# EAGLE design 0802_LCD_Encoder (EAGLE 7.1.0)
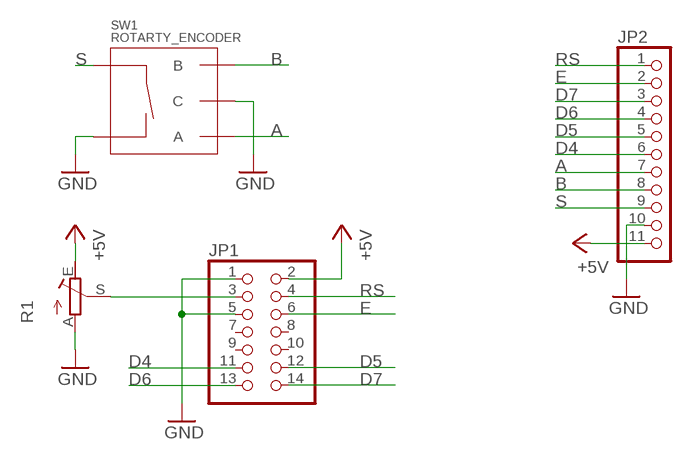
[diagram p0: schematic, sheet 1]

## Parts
JP1  PINHD-2X7  [2X07]
JP2  PINHD-1X11/90  [1X11/90]
R1  3302-TRIMMER  [3302-TRIMMER]
SW1  ROTARTY_ENCODER  [ROTARY_ENC_PLAIN]

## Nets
+5V: JP1.2 JP2.11 R1.E
A: JP2.7 SW1.A
B: JP2.8 SW1.B
D4: JP1.11 JP2.6
D5: JP1.12 JP2.5
D6: JP1.13 JP2.4
D7: JP1.14 JP2.3
E: JP1.6 JP2.2
GND: JP1.1 JP1.5 JP2.10 R1.A SW1.C SW1.SW-
RS: JP1.4 JP2.1
S: JP2.9 SW1.SW+
V0: JP1.3 R1.S
Unconnected: JP1.7 JP1.8 JP1.9 JP1.10

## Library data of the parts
JP1 = pinhead:PINHD-2X7: PIN HEADER
JP2 = pinhead:PINHD-1X11: PIN HEADER
R1 = 1Axel:3302-TRIMMER
SW1 = SparkFun-Electromechanical:ROTARTY_ENCODER: Simple no LED rotary encoder Example: COM-09117

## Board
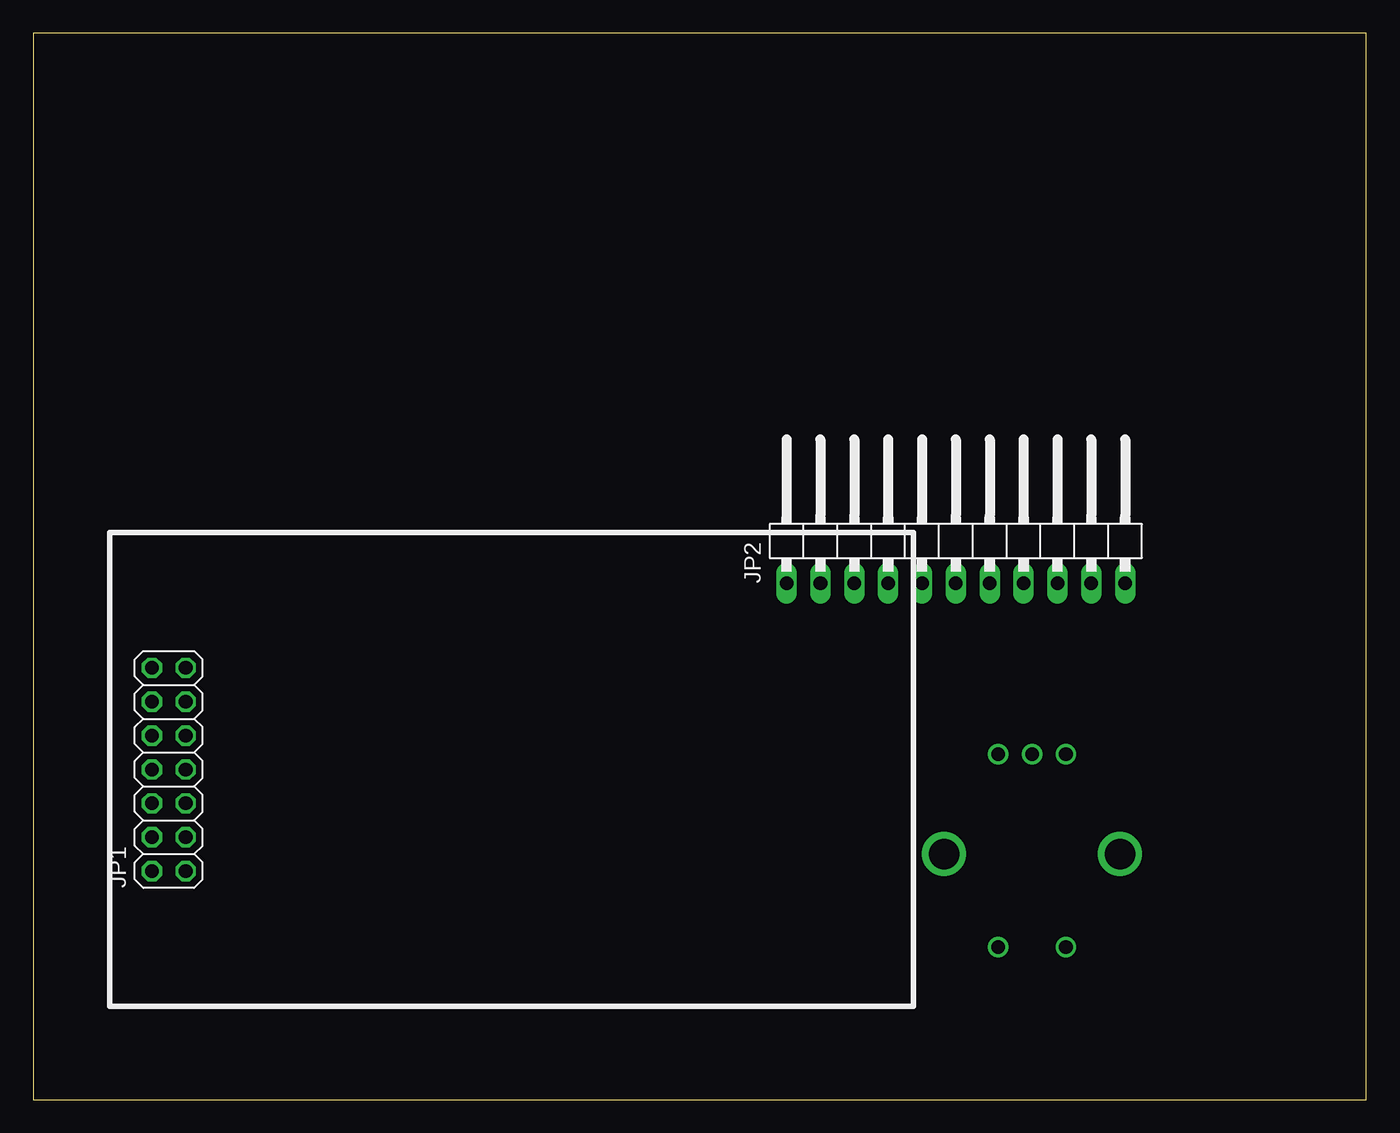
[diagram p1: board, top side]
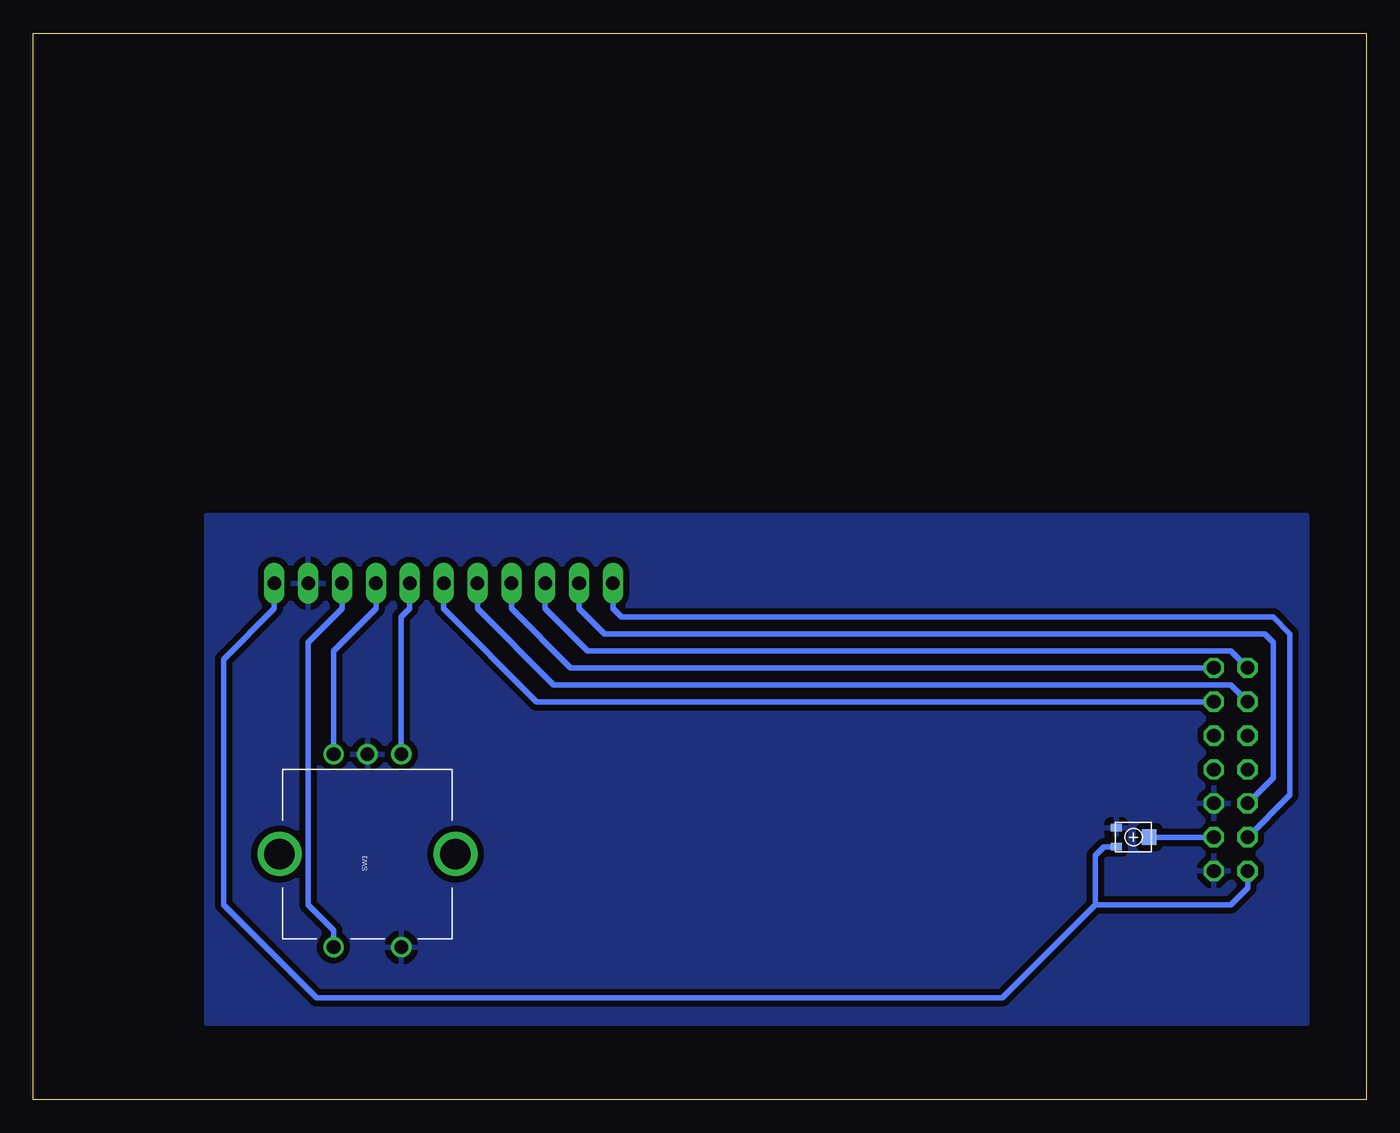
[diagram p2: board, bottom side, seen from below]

Size 100 x 80 mm. Coordinates in mm from the lower left corner, seen from the top.
Outline: 0,0 100,0 100,80 0,80 0,0
Copper layers (1*16): Top 0.035mm / dielectric 1.5mm / Bottom 0.035mm
Design rules "default *": minimum track width 10mil, minimum drill 24mil, track to track 0.4mm, track to pad 8mil, pad to pad 8mil, via to via 8mil, smd to smd 8mil, copper to edge 40mil, drill to drill 8mil, minimum pad ring 10mil, minimum via ring 8mil, stop-mask expansion 4mil, vias tented up to drill 0mil, thermal gap 20mil

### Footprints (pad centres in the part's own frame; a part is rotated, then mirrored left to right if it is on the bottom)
2X07 = drill 1.016 octagon: 1 -7.62,-1.27; 2 -7.62,1.27; 3 -5.08,-1.27; 4 -5.08,1.27; 5 -2.54,-1.27; 6 -2.54,1.27; 7 0,-1.27; 8 0,1.27; 9 2.54,-1.27; 10 2.54,1.27; 11 5.08,-1.27; 12 5.08,1.27; 13 7.62,-1.27; 14 7.62,1.27
1X11/90 = drill 1.016 long: 1 -12.7,-3.81; 2 -10.16,-3.81; 3 -7.62,-3.81; 4 -5.08,-3.81; 5 -2.54,-3.81; 6 0,-3.81; 7 2.54,-3.81; 8 5.08,-3.81; 9 7.62,-3.81; 10 10.16,-3.81; 11 12.7,-3.81
3302-TRIMMER = smd 0.572 x 0.813: A -0.714,-1.27; E 0.714,-1.27 | smd 1.194 x 1.092: S 0,1.191
ROTARY_ENC_PLAIN = drill 1.016: A 7.493,-2.54; B 7.493,2.54; C 7.493,0; SW+ -6.985,2.54; SW- -6.985,-2.54 | drill 2.286: P$3 0,6.604; P$4 0,-6.604

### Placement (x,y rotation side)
JP1  10.16,24.77 90 top
JP2  69.22,42.55 0 top
R1  17.46,19.68 270 bottom
SW1  74.93,18.41 90 bottom

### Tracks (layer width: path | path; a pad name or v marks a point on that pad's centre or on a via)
+5V
  Bottom 0.406: JP2.11 81.92,36.83 85.72,33.02 85.72,14.61 78.74,7.62 27.3,7.62 20.32,14.61 | R1.E 19.68,18.97 20.32,18.34 20.32,14.61 | JP1.2 8.89,15.88 10.16,14.61 20.32,14.61
A
  Bottom 0.406: SW1.A 72.39,36.2 71.75,36.83 JP2.7
B
  Bottom 0.406: SW1.B 77.47,33.66 74.3,36.83 JP2.8
D4
  Bottom 0.406: JP1.11 62.23,29.84 69.22,36.83 JP2.6
D5
  Bottom 0.406: JP1.12 10.16,31.11 60.96,31.11 66.67,36.83 JP2.5
D6
  Bottom 0.406: JP1.13 59.69,32.38 64.14,36.83 JP2.4
D7
  Bottom 0.406: JP1.14 10.16,33.66 58.42,33.66 61.59,36.83 JP2.3
E
  Bottom 0.406: JP1.6 6.99,24.13 6.99,34.29 7.62,34.92 57.15,34.92 59.05,36.83 JP2.2
GND
  pour Bottom (isolate 0.457): 4.45,5.71 87,5.71 87,43.81 4.45,43.81
RS
  Bottom 0.406: JP1.4 5.71,22.86 5.71,34.92 6.99,36.2 55.88,36.2 56.52,36.83 JP2.1
S
  Bottom 0.406: SW1.SW+ 77.47,12.7 79.38,14.61 79.38,34.29 76.83,36.83 JP2.9
V0
  Bottom 0.406: JP1.3 R1.S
